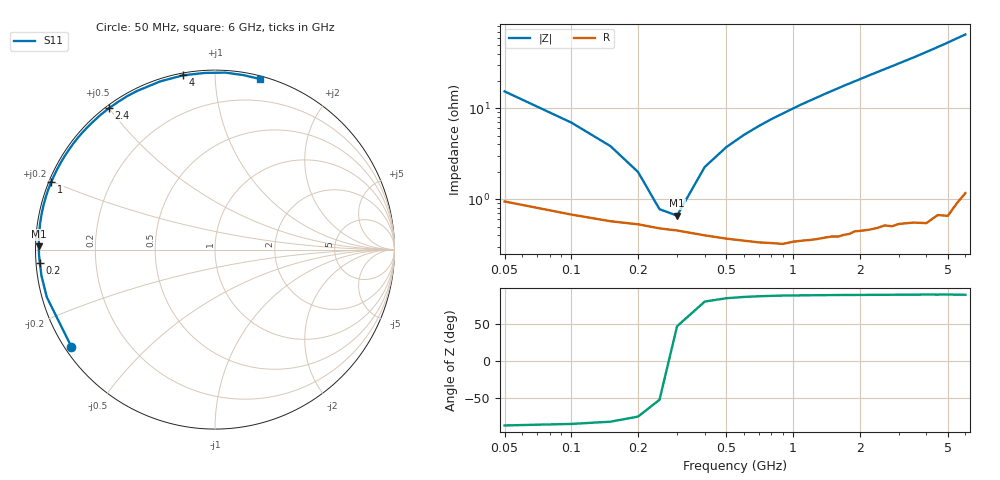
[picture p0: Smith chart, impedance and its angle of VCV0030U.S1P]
! Infineon Technologies  Discrete & RF Semiconductors
! BBY 56-03
! Si Tuning Diode in SOD323
! VR =
! S-Parameters:  June  1999
# GHz  S  MA  R  50
!  f  S11
! GHz  MAG  ANG
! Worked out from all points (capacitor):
!   34 points, 50 MHz to 6 GHz, reference 50 ohm
!   read as one part to ground: C = 200 pF near 50 MHz
!   lowest |Z| = 659 mohm at 300 MHz (marker M1)
!   series resonance near 278 MHz, so ESL is about 1.6 nH
!   S11 on the Smith chart (normalised r, x): 50 MHz: 0.02, -0.31; 200 MHz: 0.01, -0.04; 1 GHz: 0.01, +0.20; 2.4 GHz: 0.01, +0.50; 4 GHz: 0.01, +0.83; 6 GHz: 0.02, +1.30
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0.05  0.9661 -145.9
0.1  0.9738 -164.2
0.15  0.9775 -171.3
0.2  0.9791 -175.6
0.25  0.9811 -178.6
0.3  0.9821 178.9
0.4  0.9842 174.9
0.5  0.9855 171.5
0.6  0.9863 168.4
0.8  0.9872 162.7
1  0.987 157.5
1.1  0.9868 154.9
1.3  0.9864 150.1
1.4  0.9861 147.7
1.6  0.9861 143.2
1.7  0.9857 140.9
1.9  0.9848 136.7
2.2  0.9849 130.6
2.4  0.9847 126.8
2.6  0.9842 123.1
2.8  0.9851 119.6
3  0.9848 116.1
3.5  0.9856 108.0
4  0.9872 100.3
4.5  0.986 93.2
5  0.9877 86.7
5.5  0.985 80.5
6  0.9828 75.1
